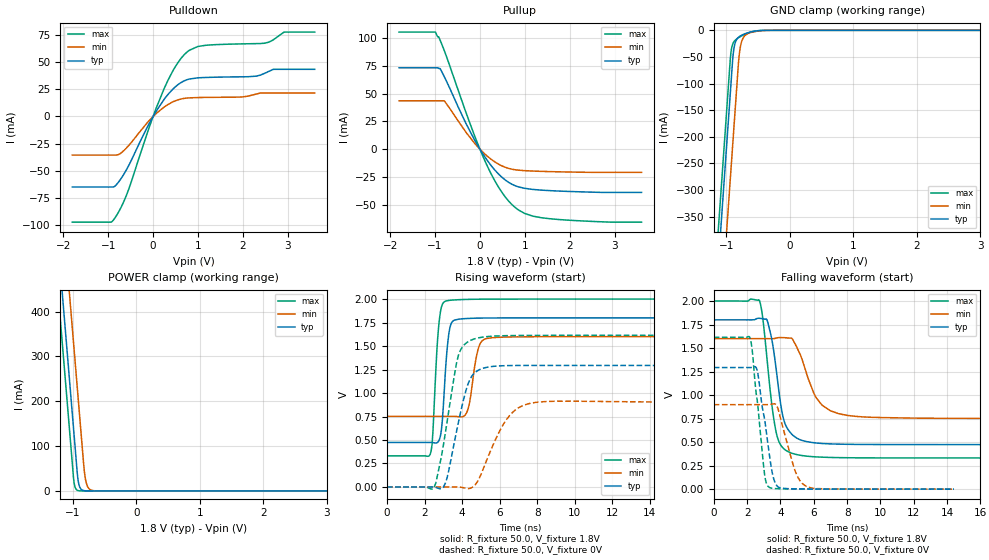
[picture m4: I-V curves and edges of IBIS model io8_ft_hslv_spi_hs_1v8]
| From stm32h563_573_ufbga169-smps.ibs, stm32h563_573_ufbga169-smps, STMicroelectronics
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[Model]   io8_ft_hslv_spi_hs_1v8
Model_type I/O
Polarity   Non-Inverting
Enable   Active-Low
| CAP_THRESHOLD on pad IOFT is "UDTCAPC" :
| Rising=20.0% of vddiom   Falling=80.0% of vddiom
| C_comp min and max val. don't necessarily correlate with the min and max pvt
| but are the smallest and greatest pad capacitance found.
| var   typ   min   max
C_comp   4.56172pF  4.45460pF  4.74984pF
|C_comp_pullup   2.85870pF  2.67900pF  2.77965pF
|C_comp_pulldown   1.70302pF  1.77560pF  1.97019pF
Vinl = 480.0mV
Vinh = 1.4V
Vmeas = 900.0mV   | Reference voltage for timing measurements
Cref  = 50.0pF   | Timing specification test load capacitance value
Rref  = 100.0MOhm   | Timing specification test load resistance value
Vref  = 900.0mV   | Timing specification test load voltage
[Model Spec]
| TIME_THRESHOLD on pin ZIV11 is "CMOS" :
| Rising=40.0% of vdd   Falling=60.0% of vdd
Vinl 703.80000mV 631.80000mV 784.80000mV
Vinh 1.06220V 937.20000mV 1.16620V
| variable   typ   min   max
[Temperature Range] 25.0 125.0 -40.0
| variable   typ   min   max
[Voltage Range] 1.8V 1.6V 2.0V
| variable   typ   min   max
[POWER Clamp Reference] 1.8V 1.6V 2.0V
| variable   typ   min   max
[GND Clamp Reference] 0V 0V 0V
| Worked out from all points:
|   slope of the pulldown table from 0 to 0.27 V, typ, clamps not added: 15.8 ohm
|   slope of the pullup table from 0 to 0.27 V, typ, clamps not added: 17.1 ohm
|   GND clamp passes 1 mA (typ) near -0.52 V on its own axis
|   POWER clamp passes 1 mA (typ) near -0.84 V on its own axis
|   rising waveform, R_fixture 50.0, V_fixture 1.8V: 20-80 % time 277ps typ, 391ps min, 268ps max; typ from 0.474 V to 1.8 V
|   falling waveform, R_fixture 50.0, V_fixture 1.8V: 20-80 % time 658ps typ, 1.18ns min, 642ps max; typ from 1.8 V to 0.474 V
|   rising waveform, R_fixture 50.0, V_fixture 0V: 20-80 % time 844ps typ, 1.27ns min, 783ps max; typ from 0 V to 1.29 V
|   falling waveform, R_fixture 50.0, V_fixture 0V: 20-80 % time 634ps typ, 860ps min, 544ps max; typ from 1.29 V to 0 V
[POWER Clamp]
-1.8V     1.518A     1.709A     1.407A
-1.23V    548.8mA    740.2mA    437.5mA
-1.16V    429.8mA    621.2mA    318.5mA
-1.05V    242.8mA    434.2mA    131.5mA
-980mV    123.8mA    315.2mA    17.95mA
-930mV    38.81mA    230.2mA    1.49mA
-910mV    17.82mA    196.2mA    550.8uA
-890mV    8.18mA     162.2mA    203.5uA
-810mV    363.5uA    33.6mA     3.797uA
-770mV    76.62uA    10.47mA    518.8nA
-710mV    7.417uA    1.822mA    26.38nA
3.6V      0A         0A         0A
[GND Clamp]
-1.8V     -1.581A    -1.742A    -1.516A
-1.24V    -628.8mA   -789.9mA   -564.1mA
-1.05V    -305.8mA   -466.9mA   -241.1mA
-940mV    -118.8mA   -279.9mA   -54.1mA
-930mV    -101.8mA   -262.9mA   -41.86mA
-900mV    -51.51mA   -211.9mA   -25.34mA
-880mV    -32.22mA   -177.9mA   -21mA
-810mV    -13.02mA   -59.5mA    -13.82mA
-770mV    -9.8mA     -24.99mA   -11mA
-680mV    -5.275mA   -7.288mA   -5.917mA
-400mV    -107uA     -349.1uA   -42.51uA
3.6V      5.392nA    968.2nA    261.3pA
| variable   typ   min   max
[Pullup Reference] 1.8V 1.6V 2.0V
| variable   typ   min   max
[Pulldown Reference] 0V 0V 0V
[Pullup]
-1.8V     73.29mA    43.57mA    105.5mA
-990mV    73.29mA    43.57mA    105.5mA
-920mV    72.69mA    43.57mA    101.3mA
-880mV    72.17mA    43.57mA    97.57mA
-790mV    65.04mA    43.33mA    88.44mA
-310mV    23.12mA    15.21mA    32.96mA
120mV     -7.55mA    -4.729mA   -11.26mA
460mV     -24.15mA   -14.46mA   -37.06mA
800mV     -33.16mA   -18.65mA   -53.01mA
1.18V     -36.29mA   -19.75mA   -60.37mA
1.56V     -37.38mA   -20.24mA   -62.7mA
3.6V      -38.97mA   -20.89mA   -65.81mA
[Pulldown]
-1.8V     -65.02mA   -35.56mA   -97.42mA
-940mV    -65.02mA   -35.56mA   -97.42mA
-850mV    -64.17mA   -35.56mA   -93.5mA
-570mV    -47.32mA   -28.01mA   -70.04mA
-120mV    -9.088mA   -5.279mA   -14.07mA
250mV     16.04mA    8.832mA    26.05mA
550mV     29.17mA    15.25mA    49.41mA
780mV     34.17mA    17.07mA    60.14mA
1.18V     35.97mA    17.56mA    65.65mA
2.49V     39.87mA    21.59mA    67.54mA
2.92V     43.47mA    21.59mA    77.77mA
3.6V      43.47mA    21.59mA    77.77mA
[Ramp]
dV/dt_r 775.79066mV/842.08425ps 539.42446mV/1.26972ns 968.30971mV/780.95088ps
dV/dt_f 795.78493mV/657.69852ps 508.93601mV/1.15231ns 1.00099V/640.62856ps
R_load = 50.0
| Removed startup time: 0s 0s 0s  .
| Removed end time: 14.4ns.
[Rising Waveform]
R_fixture   = 50.0
V_fixture   = 1.8V
V_fixture_min = 1.6V
V_fixture_max = 2.0V
0s        473.7mV    751.7mV    331.7mV
2.3ns     474mV      751.7mV    346.9mV
2.45ns    472.2mV    751.7mV    593.9mV
2.75ns    486.8mV    751.9mV    1.703V
2.9ns     607mV      751.9mV    1.916V
3.1ns     1.191V     752mV      1.976V
3.45ns    1.751V     752.3mV    1.989V
4.25ns    1.793V     794.2mV    1.996V
5.2ns     1.798V     1.573V     1.999V
14.4ns    1.8V       1.6V       2V
| Removed startup time: 0s 0s 0s  .
| Removed end time: 24.4ns.
[Falling Waveform]
R_fixture   = 50.0
V_fixture   = 1.8V
V_fixture_min = 1.6V
V_fixture_max = 2.0V
0s        1.8V       1.6V       2V
2.75ns    1.816V     1.6V       2.002V
2.95ns    1.812V     1.6V       1.803V
3.2ns     1.797V     1.6V       1.376V
3.75ns    1.266V     1.606V     599.3mV
4.15ns    772.1mV    1.611V     439.1mV
4.65ns    590.1mV    1.606V     384.3mV
6.15ns    490.8mV    970.7mV    343.1mV
7.5ns     478.6mV    802mV      335.3mV
24.4ns    473.7mV    751.8mV    331.7mV
| Removed startup time: 0s 0s 0s  .
| Removed end time: 24.3ns.
[Rising Waveform]
R_fixture   = 50.0
V_fixture   = 0V
V_fixture_min = 0V
V_fixture_max = 0V
0s        134.7nV    547nV      93.85nV
2.5ns     -524.9uV   -17.24uV   -10.08mV
2.8ns     -18.74mV   -8.69uV    227mV
3.1ns     35.25mV    -42.3uV    563.1mV
3.8ns     682.5mV    -316.2uV   1.398V
4.2ns     1.022V     -12.94mV   1.529V
4.6ns     1.201V     5.438mV    1.572V
6.3ns     1.291V     698.7mV    1.61V
7.6ns     1.293V     888.8mV    1.613V
24.3ns    1.293V     899.1mV    1.614V
| Removed startup time: 0s 0s 0s  .
| Removed end time: 14.4ns.
[Falling Waveform]
R_fixture   = 50.0
V_fixture   = 0V
V_fixture_min = 0V
V_fixture_max = 0V
0s        1.293V     898.3mV    1.614V
2.15ns    1.293V     898.3mV    1.618V
2.3ns     1.295V     898.3mV    1.487V
2.6ns     1.265V     898.3mV    953.1mV
3.05ns    745mV      898.2mV    155.1mV
3.3ns     412.9mV    898.9mV    23.05mV
3.8ns     33.94mV    879.7mV    5.33mV
4.9ns     3.282mV    185.8mV    2.205mV
5.6ns     1.929mV    25.04mV    1.433mV
14.4ns    59.82uV    216.7uV    15.22uV
